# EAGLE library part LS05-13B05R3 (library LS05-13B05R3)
AC DC CONVERTER,5W,5VDC Source: Datasheet
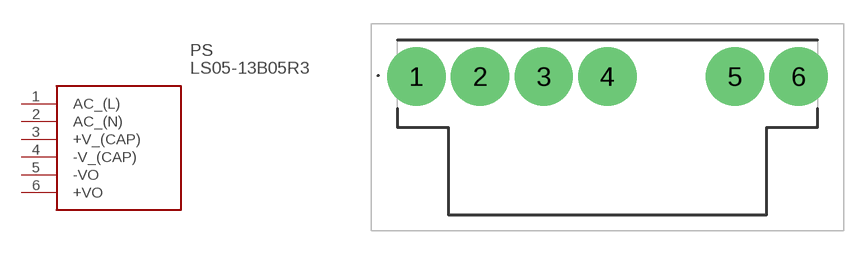
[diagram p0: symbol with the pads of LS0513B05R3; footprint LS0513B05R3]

Designator prefix PS

## LS05-13B05R3 (Description: AC DC CONVERTER,5W,5VDC; Height: 15.73mm; Manufacturer_Name: Morunsun; Manufacturer_Part_Number: LS05-13B05R3)  [LS0513B05R3]
1  AC_(L)
2  AC_(N)
3  +V_(CAP)
4  -V_(CAP)
5  -VO
6  +VO

## Footprint LS0513B05R3 (pad centres in mm)
LS05-13B05R3-2
drill 2.44 pad 3.66: 1 0,0; 2 4,0; 3 8,0; 4 12,0; 5 20,0; 6 24,0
